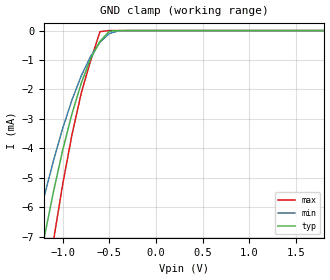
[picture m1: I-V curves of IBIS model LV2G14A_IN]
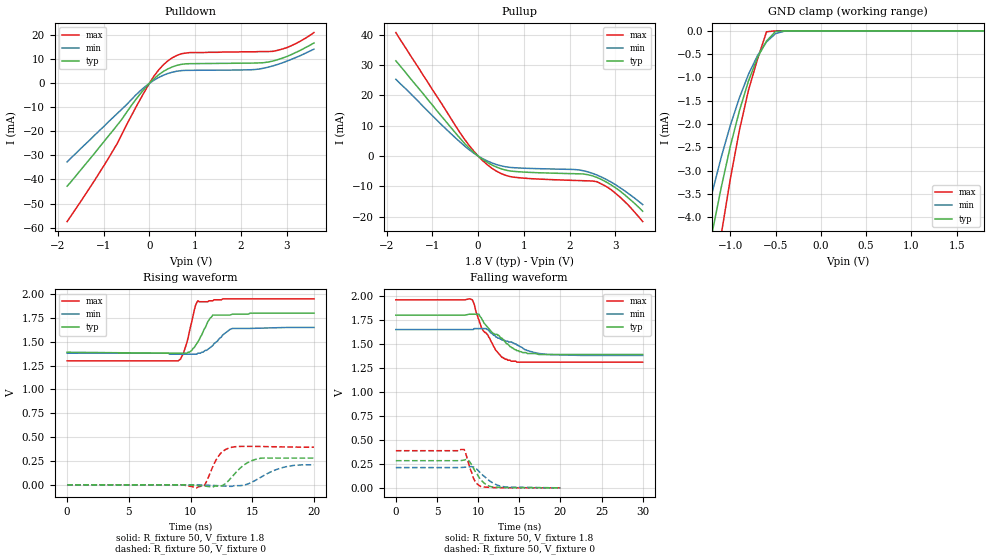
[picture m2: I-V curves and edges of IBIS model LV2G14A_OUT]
|/_/_/_/_/_/_/_/_/_/_/_/_/_/_/_/_/_/_/_/_/_/_/_/_/_/_/_/_/_/_/_/_/_/_/_/_/_/
|   Renesas Electronics Corp.
|   Multi Purpose Semiconductor Digital IC Design Group
|   IBIS Model of HD74LV2G14A
|   1.8V Triple Inverters with Schmitt-trigger Inputs,
|   SSOP-8(8pin) Package
|   History
|   V1.0   April   1, 2003   : First release.
|/_/_/_/_/_/_/_/_/_/_/_/_/_/_/_/_/_/_/_/_/_/_/_/_/_/_/_/_/_/_/_/_/_/_/_/_/_/
[IBIS Ver]   2.1
[Comment Char]  |_char
[File name]   l2g14s1.ibs
[File Rev]   1.1
[Date]   April 1, 2003
[Source]   Data created from SPICE simulations at
|   Renesas Electronics Corp.
[Notes]   RLC value of the Package is determined by assuming typical
|   conditions.
[Disclaimer]   This information is for modeling purposes only, and is not
|   guaranteed.
[Copyright]   Copyright 2003, Renesas Electronics Corp.,
|   All Rights Reserved.
|   Component  HD74LV2G14A
[Component]   HD74LV2G14A
[Manufacturer]  Renesas Electronics Corp.
[Package]
|   typ   min   max
R_pkg   0.099   0.095   0.102
L_pkg   1.740nH   1.680nH   1.790nH
C_pkg   0.140pF   0.140pF   0.150pF
[Pin]   signal_name   model_name   R_pin   L_pin   C_pin
1   1A   LV2G14A_IN   0.102   1.780nH   0.140pF
2   3Y   LV2G14A_OUT   0.097   1.710nH   0.150pF
3   2A   LV2G14A_IN   0.095   1.680nH   0.150pF
4   GND   GND   0.102   1.790nH   0.140pF
5   2Y   LV2G14A_OUT   0.101   1.790nH   0.140pF
6   3A   LV2G14A_IN   0.097   1.710nH   0.150pF
7   1Y   LV2G14A_OUT   0.097   1.710nH   0.150pF
8   VCC   POWER   0.102   1.790nH   0.140pF
| Models and submodels in the file (2): LV2G14A_IN (Input), LV2G14A_OUT (Output)
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|   Model  LV2G14A_IN
[Model]   LV2G14A_IN
Model_type  Input
Vinl = 0.54V
Vinh = 1.26V
| variable   typ   min   max
C_comp   2.85pF   2.75pF   2.95pF
| variable   typ   min   max
[Temperature range]   25   85   -40
| variable   typ   min   max
[Voltage range]   1.8V   1.65V   1.95V
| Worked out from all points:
|   GND clamp passes 1 mA (typ) near -0.71 V on its own axis
[GND Clamp]
|   Voltage   I(typ)   I(min)   I(max)
-1.8V     -19.4mA    -15.4mA    -25.6mA
-1.3V     -8.81mA    -7.02mA    -11.6mA
-1.2V     -7.07mA    -5.66mA    -9.31mA
-1.1V     -5.49mA    -4.43mA    -7.16mA
-1V       -4.06mA    -3.32mA    -5.22mA
-900mV    -2.82mA    -2.35mA    -3.53mA
-800mV    -1.78mA    -1.53mA    -2.11mA
-700mV    -950uA     -877uA     -1.02mA
-600mV    -366uA     -393uA     -35.6uA
-500mV    -21.6uA    -99uA      -429nA
-400mV    -422nA     -10.2uA    -2.45nA
1.8V      3.69pA     25.5pA     3.6pA
|   Model  LV2G14A_OUT
[Model]   LV2G14A_OUT
Model_type  Output
Polarity   Inverting
Vmeas = 0.9V
| variable   typ   min   max
C_comp   5.35pF   5.25pF   5.45pF
| variable   typ   min   max
[Temperature range]   25   85   -40
| variable   typ   min   max
[Voltage range]   1.8V   1.65V   1.95V
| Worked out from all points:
|   slope of the pulldown table from 0 to 0.27 V, typ, clamps not added: 60.6 ohm
|   slope of the pullup table from 0 to 0.27 V, typ, clamps not added: 101 ohm
|   GND clamp passes 1 mA (typ) near -0.78 V on its own axis
|   rising waveform, R_fixture 50, V_fixture 1.8: 20-80 % time 980ps typ, 1.32ns min, 733ps max; typ from 1.39 V to 1.8 V
|   rising waveform, R_fixture 50, V_fixture 0: 20-80 % time 1.35ns typ, 1.96ns min, 905ps max; typ from 0 V to 0.28 V
|   falling waveform, R_fixture 50, V_fixture 1.8: 20-80 % time 3.16ns typ, 4.08ns min, 2.33ns max; typ from 1.8 V to 1.39 V
|   falling waveform, R_fixture 50, V_fixture 0: 20-80 % time 1.34ns typ, 1.84ns min, 913ps max; typ from 0.283 V to 0 V
[Pullup]
|   Voltage   I(typ)   I(min)   I(max)
-1.8V     31.4mA     25.3mA     40.7mA
-400mV    5.92mA     4.69mA     7.77mA
-100mV    1.26mA     991uA      1.71mA
200mV     -2.09mA    -1.62mA    -2.86mA
500mV     -4.2mA     -3.22mA    -5.75mA
800mV     -5.08mA    -3.86mA    -7.01mA
2.1V      -5.82mA    -4.43mA    -8.04mA
2.4V      -6.15mA    -5.21mA    -8.18mA
2.6V      -7.07mA    -6.27mA    -8.47mA
2.9V      -9.44mA    -8.5mA     -11mA
3.1V      -11.5mA    -10.4mA    -13.5mA
3.6V      -18.2mA    -16mA      -21.6mA
[Pulldown]
|   Voltage   I(typ)   I(min)   I(max)
-1.8V     -42.8mA    -32.7mA    -57.5mA
-900mV    -22mA      -16.1mA    -31.3mA
-700mV    -17.3mA    -12.5mA    -24.9mA
-100mV    -2.12mA    -1.47mA    -3.28mA
100mV     1.89mA     1.29mA     2.99mA
400mV     5.95mA     4.05mA     9.28mA
600mV     7.46mA     5.03mA     11.6mA
900mV     8.17mA     5.4mA      12.8mA
2.2V      8.4mA      5.62mA     13.1mA
2.6V      8.86mA     6.72mA     13.2mA
3V        11.1mA     9.16mA     14.8mA
3.6V      16.8mA     14.2mA     21.1mA
[GND Clamp]
|   Voltage   I(typ)   I(min)   I(max)
-1.8V     -11.9mA    -9.46mA    -15.7mA
-1.3V     -5.4mA     -4.31mA    -7.13mA
-1.2V     -4.33mA    -3.47mA    -5.69mA
-1.1V     -3.36mA    -2.71mA    -4.37mA
-1V       -2.48mA    -2.03mA    -3.18mA
-900mV    -1.72mA    -1.44mA    -2.14mA
-800mV    -1.08mA    -936uA     -1.28mA
-700mV    -575uA     -533uA     -610uA
-600mV    -219uA     -237uA     -20.5uA
-500mV    -12.9uA    -58.6uA    -245nA
-400mV    -248nA     -6.13uA    -1.4nA
1.8V      1.91pA     29.2pA     1.8pA
[Ramp]
| variable   typ   min   max
dV/dt_r   0.174/1.442n   0.131/2.084n   0.236/904.2p
dV/dt_f   0.248/3.213n   0.164/4.184n   0.386/2.356n
R_load = 50ohms
[Rising Waveform]
R_fixture = 50
V_fixture = 1.8
V_fixture_min = 1.65
V_fixture_max = 1.95
C_fixture = 0p
|   Time   V(typ)   V(min)   V(max)
0s        1.39V      1.38V      1.3V
9ns       1.38V      1.37V      1.3V
9.4ns     1.38V      1.37V      1.37V
9.8ns     1.39V      1.37V      1.54V
10.4ns    1.46V      1.37V      1.88V
10.6ns    1.5V       1.38V      1.93V
11.4ns    1.71V      1.42V      1.92V
11.8ns    1.78V      1.46V      1.93V
13.4ns    1.79V      1.64V      1.95V
20ns      1.8V       1.65V      1.95V
[Rising Waveform]
R_fixture = 50
V_fixture = 0
C_fixture = 0p
|   Time   V(typ)   V(min)   V(max)
0s        -2.64uV    -8.9uV     -372nV
9.5ns     -2.64uV    -8.9uV     -372nV
10.5ns    -7.02mV    -901uV     -32.2mV
11.1ns    -13.2mV    -3.26mV    -9.05mV
12.2ns    -14.2mV    -9.21mV    288mV
13.1ns    46mV       -15.8mV    385mV
14.4ns    214mV      -1.04mV    403mV
15.4ns    271mV      57mV       402mV
17.5ns    280mV      182mV      397mV
20ns      280mV      210mV      394mV
[Falling Waveform]
R_fixture = 50
V_fixture = 1.8
V_fixture_min = 1.65
V_fixture_max = 1.95
C_fixture = 0p
|   Time   V(typ)   V(min)   V(max)
0s        1.8V       1.65V      1.96V
9.3ns     1.81V      1.65V      1.96V
10.1ns    1.81V      1.66V      1.75V
10.6ns    1.74V      1.66V      1.64V
11.8ns    1.61V      1.6V       1.49V
12.9ns    1.56V      1.54V      1.36V
14ns      1.47V      1.52V      1.32V
15.4ns    1.41V      1.46V      1.31V
18.4ns    1.39V      1.39V      1.31V
30ns      1.39V      1.38V      1.31V
[Falling Waveform]
R_fixture = 50
V_fixture = 0
C_fixture = 0p
|   Time   V(typ)   V(min)   V(max)
0s        283mV      211mV      387mV
7.8ns     283mV      211mV      387mV
8.3ns     290mV      214mV      400mV
8.9ns     281mV      219mV      237mV
9.5ns     194mV      214mV      88.8mV
9.9ns     140mV      189mV      40mV
10.4ns    76.6mV     146mV      11.9mV
11.4ns    16.8mV     72.2mV     5.22mV
12.7ns    5.53mV     17.7mV     716uV
20ns      -18.4uV    -39.7uV    -4.39uV
